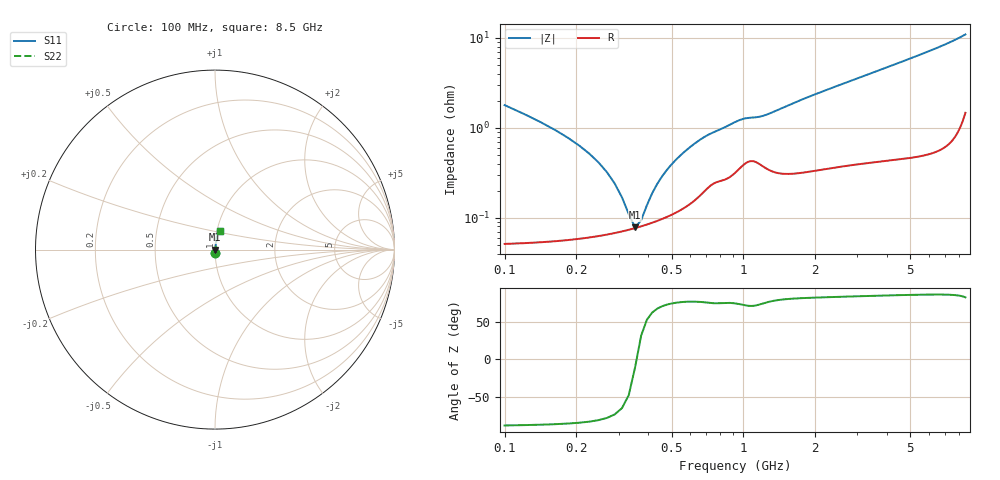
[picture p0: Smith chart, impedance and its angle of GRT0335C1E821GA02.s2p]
!Murata Part Number: GRT0335C1E821GA02
!These Parameters are Measured in Series Mode Connection
!Data Generated on Jun 19, 2026
!  o--ll--o
!Port1  Port2
!  o------o
!Operation Temp=25[degC], DC Bias Voltage=0[V]
!Freq. Start=100[MHz] Stop=9[GHz] 401[Steps]
# Hz S RI R 50
!Freq.(Hz) S11(Real) S11(Imag) S21(Real) S21(Imag) S12(Real) S12(Imag) S22(Real) S22(Imag)
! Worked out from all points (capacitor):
!   401 points, 100 MHz to 8.5 GHz, reference 50 ohm
!   read as one part in series: C = 820 pF near 142 MHz
!   lowest |Z| = 78.1 mohm at 352 MHz (marker M1)
!   series resonance near 356.8 MHz, so ESL is about 240 pH
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1e8  0.000831 -0.0179  0.9992 0.0179  0.9992 0.0179  0.000831 -0.0179
1.42e8  0.000666 -0.0115  0.9993 0.0115  0.9993 0.0115  0.000666 -0.0115
2.26e8  0.000629 -0.00513  0.9994 0.00513  0.9994 0.00513  0.000629 -0.00513
2.68e8  0.000659 -0.00315  0.9993 0.00315  0.9993 0.00315  0.000659 -0.00315
3.1e8  0.000706 -0.00153  0.9993 0.00153  0.9993 0.00153  0.000706 -0.00153
3.31e8  0.000735 -0.000814  0.9993 0.000814  0.9993 0.000814  0.000735 -0.000814
3.52e8  0.000767 -0.000145  0.9992 0.000145  0.9992 0.000145  0.000767 -0.000145
3.73e8  0.000802 0.000486  0.9992 -0.000486  0.9992 -0.000486  0.000802 0.000486
3.94e8  0.000841 0.00108  0.9992 -0.00108  0.9992 -0.00108  0.000841 0.00108
4.57e8  0.000977 0.00273  0.999 -0.00273  0.999 -0.00273  0.000977 0.00273
4.99e8  0.00109 0.00373  0.9989 -0.00373  0.9989 -0.00373  0.00109 0.00373
5.83e8  0.00139 0.00561  0.9986 -0.00561  0.9986 -0.00561  0.00139 0.00561
6.88e8  0.00203 0.00767  0.998 -0.00767  0.998 -0.00767  0.00203 0.00767
9.61e8  0.00362 0.0116  0.9964 -0.0116  0.9964 -0.0116  0.00362 0.0116
1.213e9  0.00385 0.013  0.9961 -0.013  0.9961 -0.013  0.00385 0.013
1.507e9  0.00335 0.017  0.9966 -0.017  0.9966 -0.017  0.00335 0.017
2.095e9  0.00398 0.0244  0.996 -0.0244  0.996 -0.0244  0.00398 0.0244
2.914e9  0.00503 0.034  0.995 -0.034  0.995 -0.034  0.00503 0.034
4.3e9  0.00689 0.05  0.9931 -0.05  0.9931 -0.05  0.00689 0.05
5.707e9  0.00939 0.0666  0.9906 -0.0666  0.9906 -0.0666  0.00939 0.0666
7.114e9  0.0135 0.0844  0.9865 -0.0844  0.9865 -0.0844  0.0135 0.0844
8.5e9  0.0255 0.1039  0.9745 -0.1039  0.9745 -0.1039  0.0255 0.1039
